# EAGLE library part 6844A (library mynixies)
A Burroughs 6844A nixie tube - or one of the many pin-compatible tubes
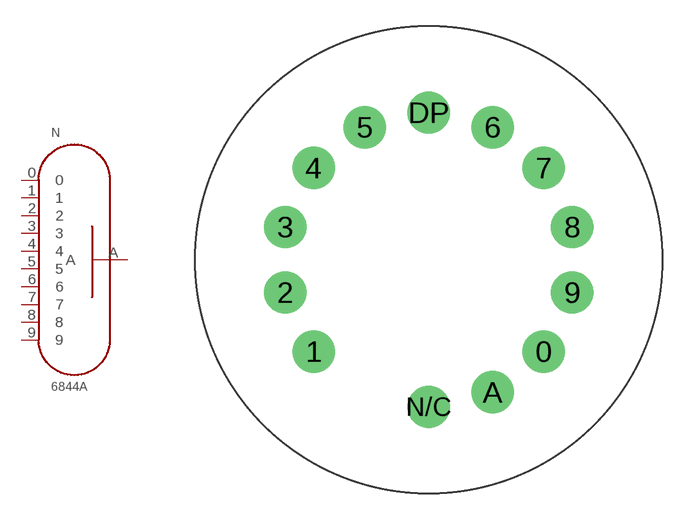
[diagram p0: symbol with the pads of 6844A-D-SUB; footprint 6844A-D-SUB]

Designator prefix N

## 6844AD-SUB  [6844A-D-SUB]
0  0  pas
1  1  pas
2  2  pas
3  3  pas
4  4  pas
5  5  pas
6  6  pas
7  7  pas
8  8  pas
9  9  pas
A  A  pas

## Footprint 6844A-D-SUB (pad centres in mm)
This footprint uses female D-SUB pins as 'sockets'.
drill 1.6: 0 6.514,-5.194; 1 -6.514,-5.194; 2 -8.122,-1.853; 3 -8.122,1.854; 4 -6.513,5.195; 5 -3.614,7.506; 6 3.615,7.506; 7 6.514,5.194; 8 8.122,1.854; 9 8.122,-1.854; A 3.615,-7.506; DP 0,8.331; N/C 0,-8.331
